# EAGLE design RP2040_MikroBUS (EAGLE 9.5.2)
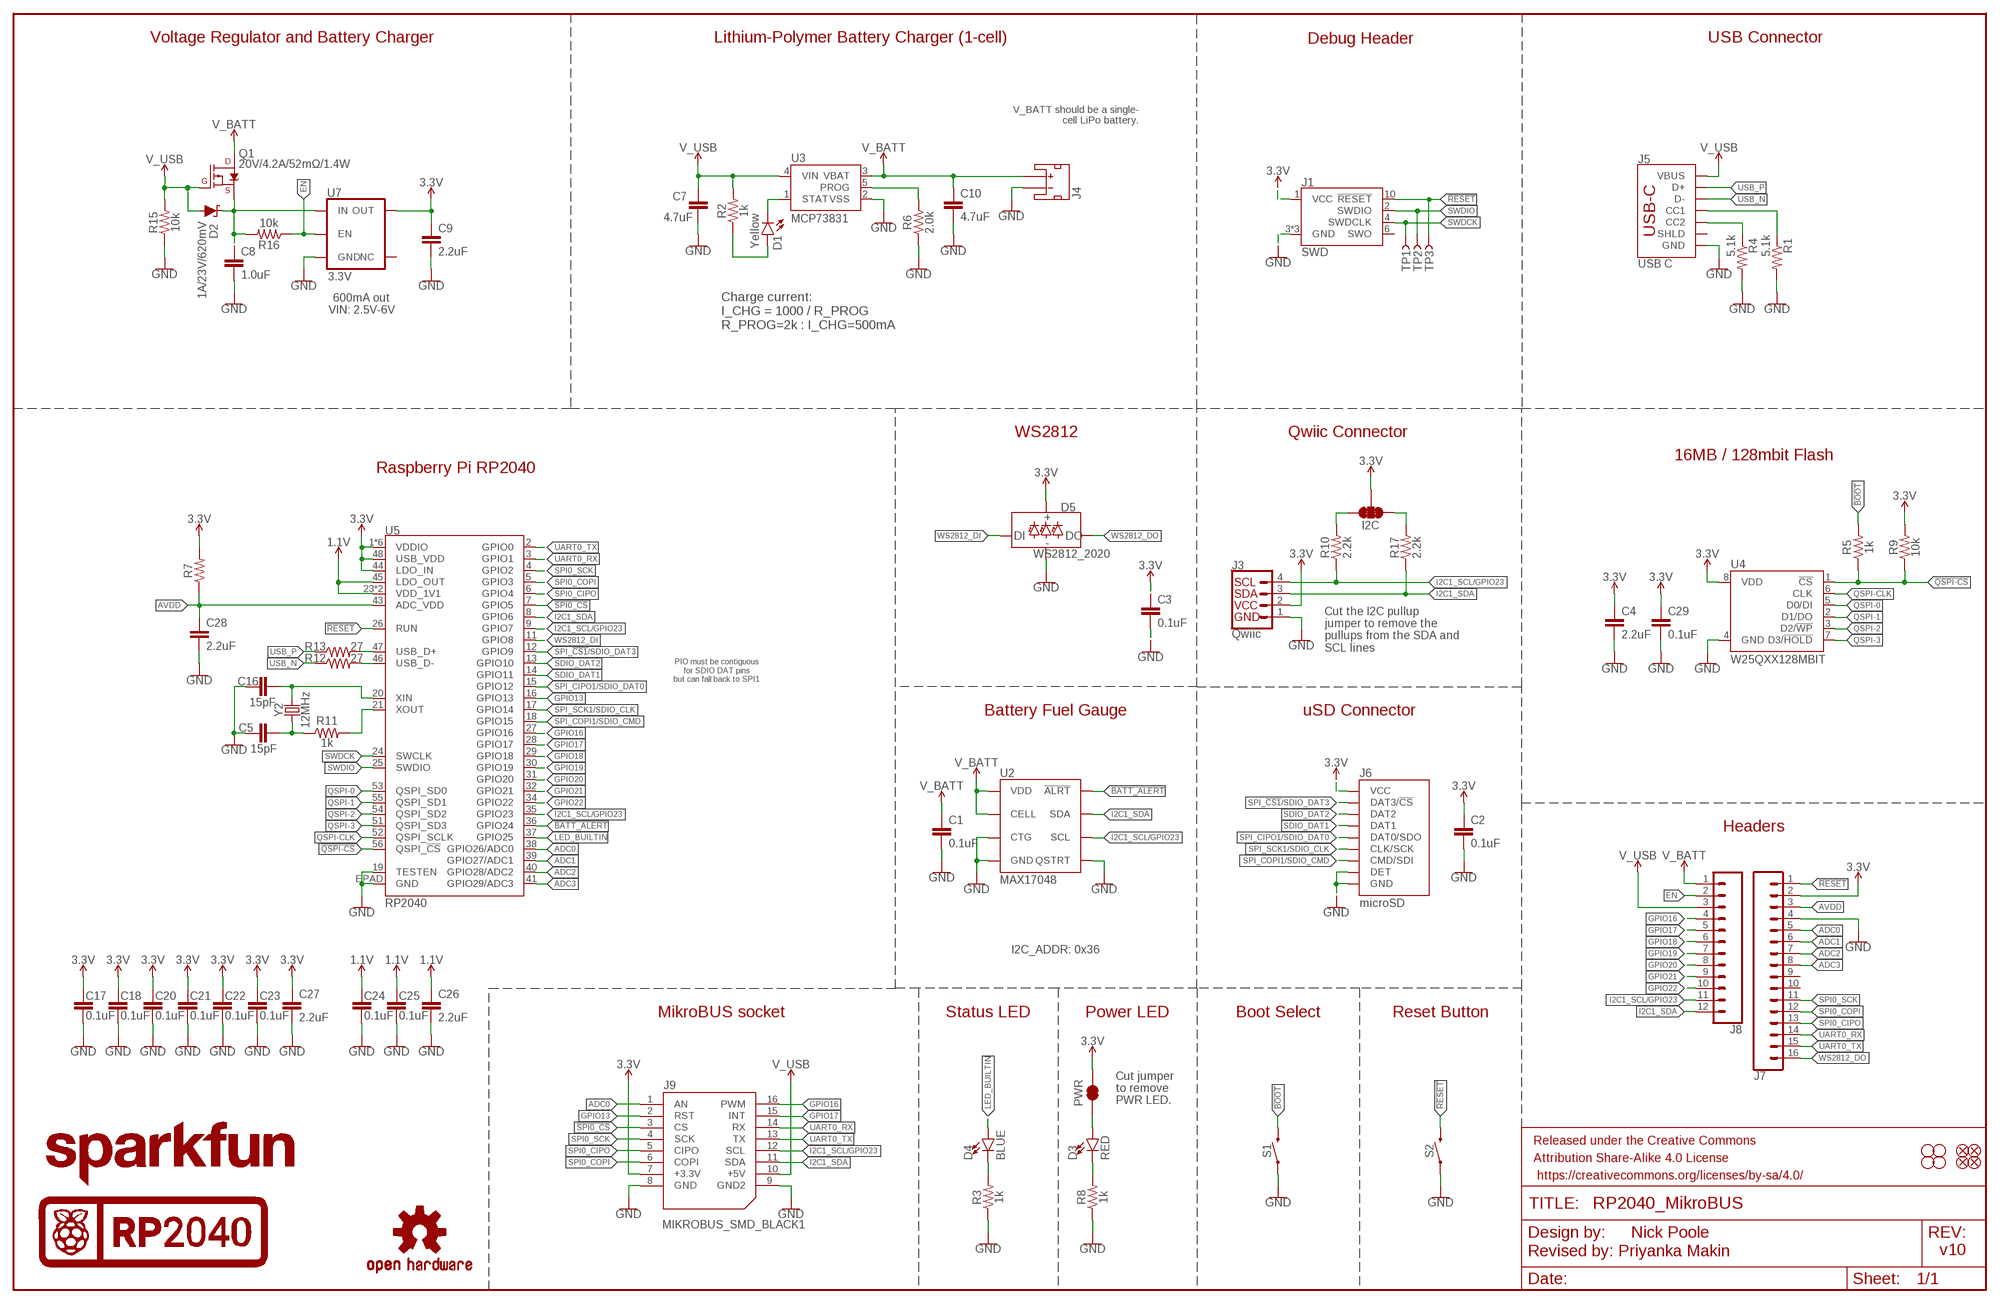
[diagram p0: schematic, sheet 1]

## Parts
C1  0.1uF  0.1UF-0402T-6.3V-10%-X7R  [0402-TIGHT]
C2  0.1uF  0.1UF-0402T-6.3V-10%-X7R  [0402-TIGHT]
C3  0.1uF  0.1UF-0402T-6.3V-10%-X7R  [0402-TIGHT]
C4  2.2uF  2.2UF-0402_TIGHT-10V-10%-X5R  [0402-TIGHT]
C5  15pF  15PF-0402T-50V-5%  [0402-TIGHT]
C7  4.7uF  4.7UF-0402_TIGHT-6.3V-20%-X5R  [0402-TIGHT]
C8  1.0uF  1.0UF-0402T-16V-10%  [0402-TIGHT]
C9  2.2uF  2.2UF-0402_TIGHT-10V-10%-X5R  [0402-TIGHT]
C10  4.7uF  4.7UF-0402_TIGHT-6.3V-20%-X5R  [0402-TIGHT]
C16  15pF  15PF-0402T-50V-5%  [0402-TIGHT]
C17  0.1uF  0.1UF-0402T-6.3V-10%-X7R  [0402-TIGHT]
C18  0.1uF  0.1UF-0402T-6.3V-10%-X7R  [0402-TIGHT]
C20  0.1uF  0.1UF-0402T-6.3V-10%-X7R  [0402-TIGHT]
C21  0.1uF  0.1UF-0402T-6.3V-10%-X7R  [0402-TIGHT]
C22  0.1uF  0.1UF-0402T-6.3V-10%-X7R  [0402-TIGHT]
C23  0.1uF  0.1UF-0402T-6.3V-10%-X7R  [0402-TIGHT]
C24  0.1uF  0.1UF-0402T-6.3V-10%-X7R  [0402-TIGHT]
C25  0.1uF  0.1UF-0402T-6.3V-10%-X7R  [0402-TIGHT]
C26  2.2uF  2.2UF-0402_TIGHT-10V-10%-X5R  [0402-TIGHT]
C27  2.2uF  2.2UF-0402_TIGHT-10V-10%-X5R  [0402-TIGHT]
C28  2.2uF  2.2UF-0402_TIGHT-10V-10%-X5R  [0402-TIGHT]
C29  0.1uF  0.1UF-0402T-6.3V-10%-X7R  [0402-TIGHT]
D1  Yellow  LED-YELLOW0603  [LED-0603]
D2  1A/23V/620mV  DIODE-SCHOTTKY-BAT20J  [SOD-323]
D3  RED  LED-RED0603  [LED-0603]
D4  BLUE  LED-BLUE0603  [LED-0603]
D5  WS2812_2020  [WS2812-2020]
FD1  FIDUCIALUFIDUCIAL  [FIDUCIAL-MICRO]
FD2  FIDUCIALUFIDUCIAL  [FIDUCIAL-MICRO]
FD3  FIDUCIALUFIDUCIAL  [FIDUCIAL-MICRO]
FD4  FIDUCIALUFIDUCIAL  [FIDUCIAL-MICRO]
FRAME1  FRAME-LEDGER  [CREATIVE_COMMONS]
H1  STAND-OFF  [STAND-OFF]
H2  STAND-OFF  [STAND-OFF]
H3  STAND-OFF  [STAND-OFF]
H4  STAND-OFF  [STAND-OFF]
I2C  JUMPER-SMT_3_2-NC_TRACE_SILK  [SMT-JUMPER_3_2-NC_TRACE_SILK]
J1  SWD  CORTEX_JTAG_DEBUG_MINIMUM_PTH  [2X5-PTH-1.27MM]
J3  Qwiic  QWIIC_CONNECTORJS-1MM  [JST04_1MM_RA]
J4  JST_2MM_MALE  [JST-2-SMD]
J5  USB C  USB_C_4-LAYER-ISOLATED  [USB-C-16P-4LAYER-ISOLATED]
J6  microSD  MICRO-SD-PUSH-PUSH-EXT-PIN  [MICROSD-EXTERNALPIN]
J7  CONN_161X16_NO_SILK  [1X16_NO_SILK]
J8  CONN_12NO_SILK  [1X12_NO_SILK]
J9  MIKROBUS_SMD_BLACK1  [MIKROBUS_SMD_BLACK]
LOGO1  OSHW-LOGOS  [OSHW-LOGO-S]
LOGO2  SFE_LOGO_NAME.1_INCH  [SFE_LOGO_NAME_.1]
PWR  JUMPER-SMT_2_NC_TRACE_SILK  [SMT-JUMPER_2_NC_TRACE_SILK]
Q1  20V/4.2A/52mΩ/1.4W  MOSFET_PCH-DMG2305UX-7  [SOT23-3]
R1  5.1k  5.1KOHM-0402T-1/16W-1%  [0402-TIGHT]
R2  1k  1KOHM-0402T-1/16W-1%  [0402-TIGHT]
R3  1k  1KOHM-0402T-1/16W-1%  [0402-TIGHT]
R4  5.1k  5.1KOHM-0402T-1/16W-1%  [0402-TIGHT]
R5  1k  1KOHM-0402T-1/16W-1%  [0402-TIGHT]
R6  2.0k  2.0KOHM-0603-1/10W-5%  [0603]
R7  200OHM-0402T-1/16W-1%  [0402-TIGHT]
R8  1k  1KOHM-0402T-1/16W-1%  [0402-TIGHT]
R9  10k  10KOHM-0402T-1/16W-1%  [0402-TIGHT]
R10  2.2k  2.2KOHM-0402T-1/16W-1%  [0402-TIGHT]
R11  1k  1KOHM-0402T-1/16W-1%  [0402-TIGHT]
R12  27  27OHM  [0402-TIGHT]
R13  27  27OHM  [0402-TIGHT]
R15  10k  10KOHM-0402T-1/16W-1%  [0402-TIGHT]
R16  10k  10KOHM-0402T-1/16W-1%  [0402-TIGHT]
R17  2.2k  2.2KOHM-0402T-1/16W-1%  [0402-TIGHT]
S1  MOMENTARY-SWITCH-SPST-SMD-5.2MM-TALL  [TACTILE_SWITCH_SMD_5.2MM]
S2  MOMENTARY-SWITCH-SPST-SMD-5.2MM-TALL  [TACTILE_SWITCH_SMD_5.2MM]
TP1  TEST-POINT3X4  [PAD.03X.04]
TP2  TEST-POINT3X4  [PAD.03X.04]
TP3  TEST-POINT3X4  [PAD.03X.04]
U2  MAX17048  MAX17048DFN8  [DFN-8]
U3  MCP73831  [SOT23-5]
U4  W25QXX128MBIT  W25QXX128MBIT-6X5-SKINNY_CENTER  [WSON-8-6X5-SKINNY_CENTERPAD]
U5  RP2040  [QFN-56]
U7  3.3V  V_REG_AP2112K-3.3V  [SOT23-5]
U$17  RASPI_RP2040_LOGO_10MM  [RASPI_RP2040_LOGO_10MM]
U$73  RASPI_RP2040_LOGO_10MM  [RASPI_RP2040_LOGO_10MM]
Y2  12MHz  CRYSTAL-12MHZ  [CRYSTAL-SMD-2X2.5MM]

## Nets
1.1V: C24.1 C25.1 C26.1 U5.23(VDD_1V1) U5.45(LDO_OUT) U5.50(VDD_1V1)
3.3V: C2.1 C3.1 C4.1 C9.1 C17.1 C18.1 C20.1 C21.1 C22.1 C23.1 C27.1 C29.1 D5.VCC I2C.2 J1.1(VCC) J3.2 J6.4(VCC) J7.2 J9.7(+3.3V) PWR.2 R7.2 R9.2 U4.8(VDD) U5.1(VDDIO) U5.10(VDDIO) U5.22(VDDIO) U5.33(VDDIO) U5.42(VDDIO) U5.44(LDO_IN) U5.48(USB_VDD) U5.49(VDDIO) U7.5(OUT)
!BATT_ALERT!: U2.5(!ALRT) U5.36(GPIO24)
!BOOT!: R5.2 S1.3
!QSPI-CS!: R5.1 R9.1 U4.1(!CS!) U5.56(QSPI_!CS!)
!RESET!: J1.10(!RESET) J7.1 S2.3 TP3.1 U5.26(RUN)
!SPI0_CS!: J9.3(CS) U5.7(GPIO5)
ADC0: J7.5 J9.1(AN) U5.38(GPIO26/ADC0)
ADC1: J7.6 U5.39(GPIO27/ADC1)
ADC2: J7.7 U5.40(GPIO28/ADC2)
ADC3: J7.8 U5.41(GPIO29/ADC3)
AVDD: C28.1 J7.3 R7.1 U5.43(ADC_VDD)
EN: J8.2 R16.1 U7.3(EN)
GND: C1.2 C2.2 C3.2 C4.2 C5.1 C7.2 C8.2 C9.2 C10.2 C16.1 C17.2 C18.2 C20.2 C21.2 C22.2 C23.2 C24.2 C25.2 C26.2 C27.2 C28.2 C29.2 D5.GND J1.3(GND) J1.5(GND) J1.9(GND) J3.1 J4.1(-) J5.GND J5.GND2(GND) J6.6(GND) J6.9(DET) J6.10(GND) J6.11(GND) J6.12(GND) J6.13(GND) J7.4 J9.8(GND) J9.9(GND2) R1.2 R3.1 R4.2 R6.1 R8.1 R15.1 S1.1 S2.1 U2.1(CTG) U2.4(GND) U2.6(QSTRT) U2.9(GND) U3.2(VSS) U4.4(GND) U5.19(TESTEN) U5.EPAD(GND) U7.2(GND)
GPIO13: J9.2(RST) U5.16(GPIO13)
GPIO16: J8.4 J9.16(PWM) U5.27(GPIO16)
GPIO17: J8.5 J9.15(INT) U5.28(GPIO17)
GPIO18: J8.6 U5.29(GPIO18)
GPIO19: J8.7 U5.30(GPIO19)
GPIO20: J8.8 U5.31(GPIO20)
GPIO21: J8.9 U5.32(GPIO21)
GPIO22: J8.10 U5.34(GPIO22)
I2C1_SCL/GPIO23: J3.4 J8.11 J9.12(SCL) R10.1 U2.7(SCL) U5.9(GPIO7) U5.35(GPIO23)
I2C1_SDA: J3.3 J8.12 J9.11(SDA) R17.1 U2.8(SDA) U5.8(GPIO6)
LED_BUILTIN: D4.A U5.37(GPIO25)
N$1: D4.C R3.2
N$2: I2C.3 R10.2
N$3: I2C.1 R17.2
N$4: R11.2 U5.21(XOUT)
N$5: C16.2 U5.20(XIN) Y2.P3
N$6: C5.2 R11.1 Y2.P1
N$7: D3.C R8.2
N$9: D1.C U3.1(STAT)
N$10: D3.A PWR.1
N$11: J5.A5(CC1) R1.1
N$12: J5.B5(CC2) R4.1
N$14: R6.2 U3.5(PROG)
N$15: C8.1 D2.C Q1.2(S) R16.2 U7.1(IN)
N$17: D1.A R2.1
QSPI-0: U4.5(D0/DI) U5.53(QSPI_SD0)
QSPI-1: U4.2(D1/DO) U5.55(QSPI_SD1)
QSPI-2: U4.3(D2/!WP!) U5.54(QSPI_SD2)
QSPI-3: U4.7(D3/!HOLD!) U5.51(QSPI_SD3)
QSPI-CLK [Clock]: U4.6(CLK) U5.52(QSPI_SCLK)
SDIO_DAT1: J6.8(DAT1) U5.14(GPIO11)
SDIO_DAT2: J6.1(DAT2) U5.13(GPIO10)
SPI0_CIPO: J7.13 J9.5(CIPO) U5.6(GPIO4)
SPI0_COPI: J7.12 J9.6(COPI) U5.5(GPIO3)
SPI0_SCK: J7.11 J9.4(SCK) U5.4(GPIO2)
SPI_!CS1!/SDIO_DAT3: J6.2(DAT3/!CS!) U5.12(GPIO9)
SPI_CIPO1/SDIO_DAT0: J6.7(DAT0/SDO) U5.15(GPIO12)
SPI_COPI1/SDIO_CMD: J6.3(CMD/SDI) U5.18(GPIO15)
SPI_SCK1/SDIO_CLK: J6.5(CLK/SCK) U5.17(GPIO14)
SWDCK: J1.4(SWDCLK) TP1.1 U5.24(SWCLK)
SWDIO: J1.2(SWDIO) TP2.1 U5.25(SWDIO)
UART0_RX: J7.14 J9.14(RX) U5.3(GPIO1)
UART0_TX: J7.15 J9.13(TX) U5.2(GPIO0)
USB_F_N: R12.2 U5.46(USB_D-)
USB_F_P: R13.2 U5.47(USB_D+)
USB_N: J5.A7(D-) J5.B7(D-) R12.1
USB_P: J5.A6(D+) J5.B6(D+) R13.1
V_BATT: C1.1 C10.1 J4.2(+) J8.1 Q1.3(D) U2.2(CELL) U2.3(VDD) U3.3(VBAT)
V_USB: C7.1 D2.A J5.VBUS1(VBUS) J5.VBUS2(VBUS) J8.3 J9.10(+5V) Q1.1(G) R2.2 R15.2 U3.4(VIN)
WS2812_DI: D5.DI U5.11(GPIO8)
WS2812_DO: D5.DO J7.16
Unconnected: J1.6(SWO) J4.NC1(PAD1) J4.NC2(PAD2) J5.SHLD1(SHLD) J5.SHLD2(SHLD) J5.SHLD3(SHLD) J5.SHLD4(SHLD) J5.SHLD5(SHLD) J5.SHLD6(SHLD) J5.SHLD7(SHLD) J5.SHLD8(SHLD) J7.9 J7.10 U7.4(NC)

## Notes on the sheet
- Voltage Regulator and Battery Charger | Lithium-Polymer Battery Charger (1-cell) | Debug Header | USB Connector
- V_BATT should be a single-
  cell LiPo battery.
- Charge current:
  I_CHG = 1000 / R_PROG
  R_PROG=2k : I_CHG=500mA
- 600mA out
  VIN: 2.5V-6V
- WS2812 | Qwiic Connector
- 16MB / 128mbit Flash
- Raspberry Pi RP2040
- Cut the I2C pullup 
  jumper to remove the 
  pullups from the SDA and 
  SCL lines
- PIO must be contiguous
  for SDIO DAT pins
  but can fall back to SPI1
- Battery Fuel Gauge | uSD Connector
- Headers
- I2C_ADDR: 0x36
- MikroBUS socket | Status LED | Power LED | Boot Select | Reset Button
- Cut jumper
  to remove
  PWR LED.
- Nick Poole
- v10
- Revised by: Priyanka Makin

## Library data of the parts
C1-C3 C17 C18 C20-C25 C29 = SparkFun-Capacitors:0.1UF: 0.1µF ceramic capacitors; PROD_ID: CAP-14993
C4 C9 C26-C28 = SparkFun-Capacitors:2.2UF: 2.2µF ceramic capacitors; PROD_ID: CAP-14232
C5 C16 = SparkFun-Capacitors:15PF: 15pF ceramic capacitors; PROD_ID: CAP-13063
C7 C10 = SparkFun-Capacitors:4.7UF: 4.7µF ceramic capacitors; PROD_ID: CAP-14240
C8 = SparkFun-Capacitors:1.0UF: 1µF ceramic capacitors; PROD_ID: CAP-12417
D1 = SparkFun-LED:LED-YELLOW: Yellow SMD LED; PROD_ID: DIO-09003
D2 = SparkFun-DiscreteSemi:DIODE-SCHOTTKY: Schottky diode; PROD_ID: DIO-11623
D3 = SparkFun-LED:LED-RED: Red SMD LED; PROD_ID: DIO-00819
D4 = SparkFun-LED:LED-BLUE: Blue SMD LED; PROD_ID: DIO-08575
D5 = SparkFun-LED:WS2812: Addressable RGB LED - 1 Wire Common names: WS2812, SK6812, Neopixel, APA-106, etc. SMD LED with built-in controller IC. Color: Red/Green/Blue SparkFun Products: LED-SMD RGB (WS2812) LED - RGB Addressable, PTH, 5mm Diffused (5 Pack) LED - RGB Addressable, PTH, 5mm Clear (5 Pack) Blynk Board -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; PROD_ID: DIO-15591
FD1-FD4 = SparkFun-Aesthetics:FIDUCIAL: Fiducial Alignment Points
FRAME1 = SparkFun-Aesthetics:FRAME-LEDGER: Schematic Frame - Ledger
H1-H4 = SparkFun-Hardware:STAND-OFF: Stand Off
I2C = SparkFun-Jumpers:JUMPER-SMT_3_2-NC_TRACE: Normally closed trace jumper (2 of 2 connections) This jumper has a trace between all three pads so they are normally closed (NC). Use a razor knife to open the connection(s). For best results follow the IPC guidelines for cutting traces: Cutout at least 0.063 mm (0.005 in). Remove all loose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
J1 = SparkFun-Connectors:CORTEX_JTAG_DEBUG_MINIMUM: Cortex Debug Connector - 10 pin Supports JTAG debug, Serial Wire debug, and Serial Wire Viewer. PTH and SMD connector options available. General Connector Information Products: PTH Connector -via Digi-Key SparkFun PSoc SparkFun T
J3 = SparkFun-Connectors:QWIIC_CONNECTOR: SparkFun I2C Standard Qwiic Connector An SMD 1mm pitch JST connector makes it easy and quick (get it? Qwiic?) to connect I2C devices to each other. The Qwiic system enables fast and solderless connection between popular platforms and various sensors and actuators. We carry 200mm, 100mm, 50mm, and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; PROD_ID: CONN-13694; VALUE: QWIIC_RIGHT_ANGLE
J4 = SparkFun-Connectors:JST_2MM_MALE: JST 2MM MALE RA CONNECTOR Two pin, compact surface mount connector. Commonly used as a battery input connection point. We really like the solid locking feeling and high current rating on these small connectors. We use these all the time as battery connectors. Mates to single-cell LiPo batteries.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; PROD_ID: CONN-11443; SF_ID: PRT-08612
J5 = SparkFun-Connectors:USB_C: USB Type C 16Pin Connector Super Speed pins not available on the 16-pin purely SMD connector so this part is best for USB 2.0 implementations. D1 and D2 are tied together enabling D+/- no matter which way the cable is plugged into the connector. The two channel configuration pins (CC1/2) are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; PROD_ID: CONN-14122; VALUE: USB Female Type C Connector
J6 = SparkFun-Connectors:MICRO-SD: microSD Socket for Transflash Various sockets for µSD. tDoc lines correctly indicate media card edge positions when inserting (unlocked, locked, depressed). NOTE: CD1 and CD2 are connected internally, and the default detect state of the socket is detect pin to ground. SparkFun Products: WAV Trigger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; PROD_ID: CONN-16110
J7 = SparkFun-Connectors:CONN_16: Multi connection point. Often used as Generic Header-pin footprint for 0.1 inch spaced/style header connections On any of the 0.1 inch spaced packages, you can populate with these: Break Away Headers - Straight (PRT-00116) Break Away Male Headers - Right Angle (PRT-00553) Female Headers (PRT-00115)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
J8 = SparkFun-Connectors:CONN_12: Multi connection point. Often used as Generic Header-pin footprint for 0.1 inch spaced/style header connections On any of the 0.1 inch spaced packages, you can populate with these: Break Away Headers - Straight (PRT-00116) Break Away Male Headers - Right Angle (PRT-00553) Female Headers (PRT-00115)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
J9 = mikroBUS_SMD_BLACK:MIKROBUS_SMD_BLACK; PROD_ID: CONN-16267
LOGO1 = SparkFun-Aesthetics:OSHW-LOGO: Open-Source Hardware (OSHW) Logo
LOGO2 = SparkFun-Aesthetics:SFE_LOGO_NAME: SparkFun Font Logo
PWR = SparkFun-Jumpers:JUMPER-SMT_2_NC_TRACE: Normally closed trace jumper
Q1 = SparkFun-DiscreteSemi:MOSFET_PCH: P-channel MOSFETs Voltage controlled devices that allow control of high current outputs. SparkFun Products: SparkFun ESP32 Thing SparkFun ESP8266 Thing SparkFun Pi Servo HAT V2 DMG2305UX-7 (20V/4.2A/SOT23-3); PROD_ID: TRANS-14388
R1 R4 = SparkFun-Resistors:5.1KOHM; PROD_ID: RES-14340
R2 R3 R5 R8 R11 = SparkFun-Resistors:1KOHM: 1kΩ resistor; PROD_ID: RES-14342
R6 = SparkFun-Resistors:2.0KOHM: 2kΩ resistor; PROD_ID: RES-08296
R7 = SparkFun-Resistors:200OHM: 200Ω resistor; PROD_ID: RES-15550
R9 R15 R16 = SparkFun-Resistors:10KOHM: 10kΩ resistor; PROD_ID: RES-14241
R10 R17 = SparkFun-Resistors:2.2KOHM: 2.2kΩ resistor; PROD_ID: RES-14341
R12 R13 = SparkFun-Resistors:27OHM: 27Ω resistor; PROD_ID: RES-15238
S1 S2 = SparkFun-Switches:MOMENTARY-SWITCH-SPST: Momentary Switch (Pushbutton) - SPST; PROD_ID: SWCH-14139
TP1-TP3 = SparkFun-Connectors:TEST-POINT: SparkFun Test Points
U2 = SparkFun-IC-Power:MAX17048: Micropower 1-Cell Li+ ModelGauge SparkFun Products Qduino Mini (DEV-13614); PROD_ID: IC-12551
U3 = SparkFun-IC-Power:MCP73831: MCP73831T Li-Ion, Li-Pol Controller Miniature single cell, fully integrated Li-Ion, Li-polymer charge management controller Datasheet SparkFun Products: SparkFun ESP32 Thing SparkFun 9DoF Razor IMU M0; PROD_ID: IC-09995
U4 = SparkFun-IC-Memory:W25QXX; PROD_ID: IC-15107
U5 = SparkFun-IC-Microcontroller:RP2040: Raspberry Pi RP2040 MCU 56-pin 32-bit Microcontroller with 264kB of SRAM and external flash support up to 16MB Getting Started with the RP2040 Dual-core ARM Cortex M0+ processor, flexible clock running up to 133 MHz 264kB of SRAM, and QSPI control of common flash memory USB 1.1 Host and Device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; PROD_ID: IC-15502
U7 = SparkFun-IC-Power:V_REG_AP2112: AP2112 - 600mA CMOS LDO Regulator w/ Enable The AP2112 is CMOS process low dropout linear regulator with enable function, the regulator delivers a guaranteed 600mA (min.) continuous load current. Features Output Voltage Accuracy: ±1.5% Output Current: 600mA (Min.) Foldback Short Current Protection: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; PROD_ID: VREG-12457
U$17 U$73 = SparkFun-Aesthetics:RASPI_RP2040_LOGO
Y2 = SparkFun-Clocks:CRYSTAL-12MHZ: 12.0MHz Crystal; PROD_ID: XTAL-15540

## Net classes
0 default: width 0 mm, drill 0 mm
2 Clock: width 0.089 mm, clearance 0.178 mm

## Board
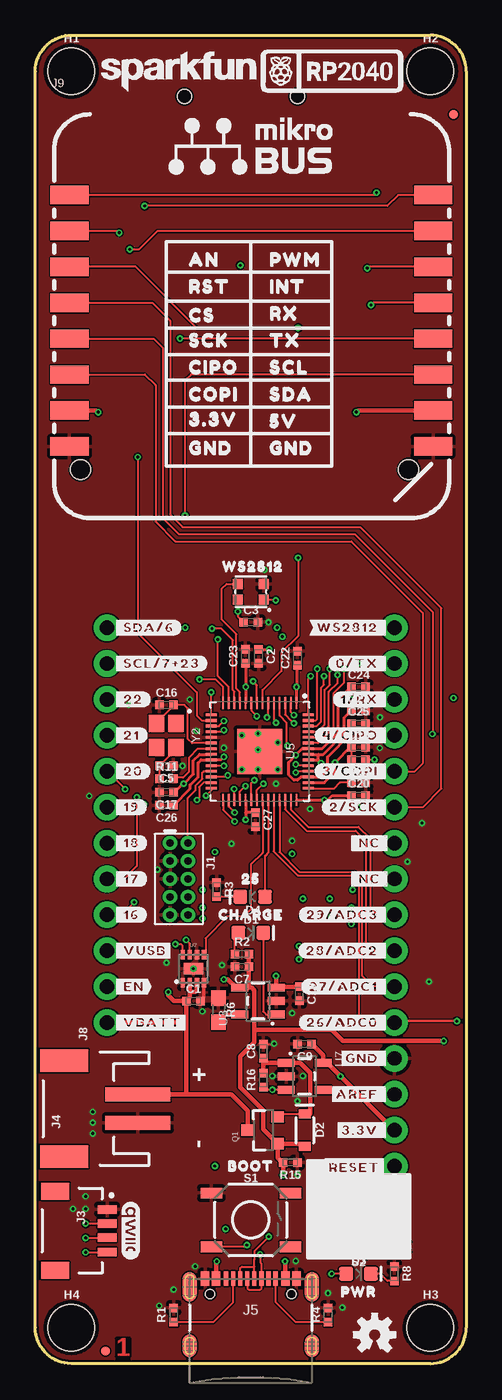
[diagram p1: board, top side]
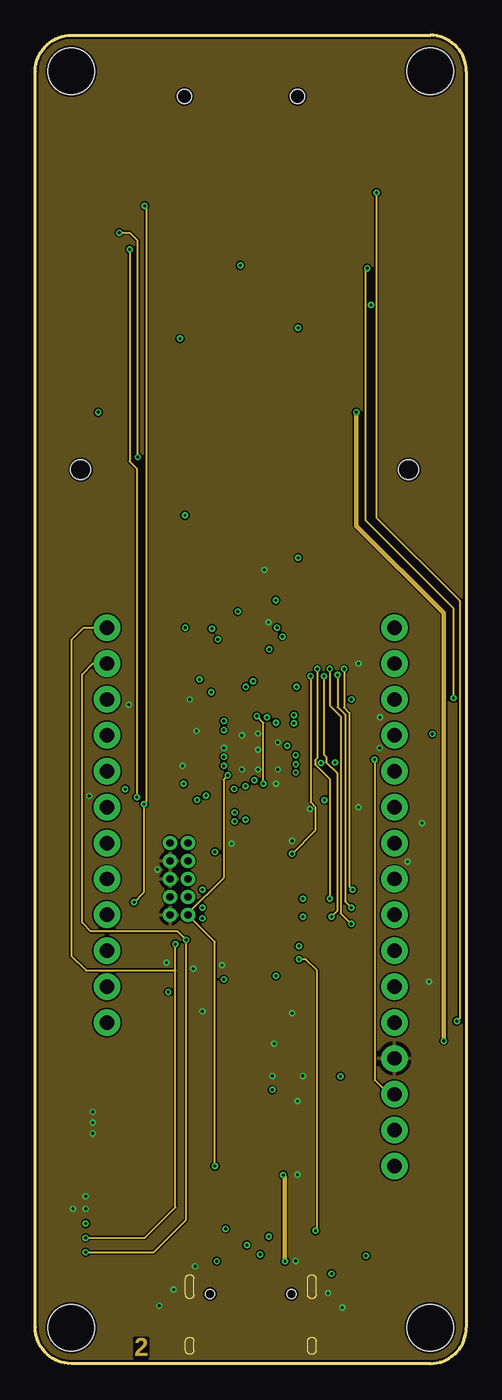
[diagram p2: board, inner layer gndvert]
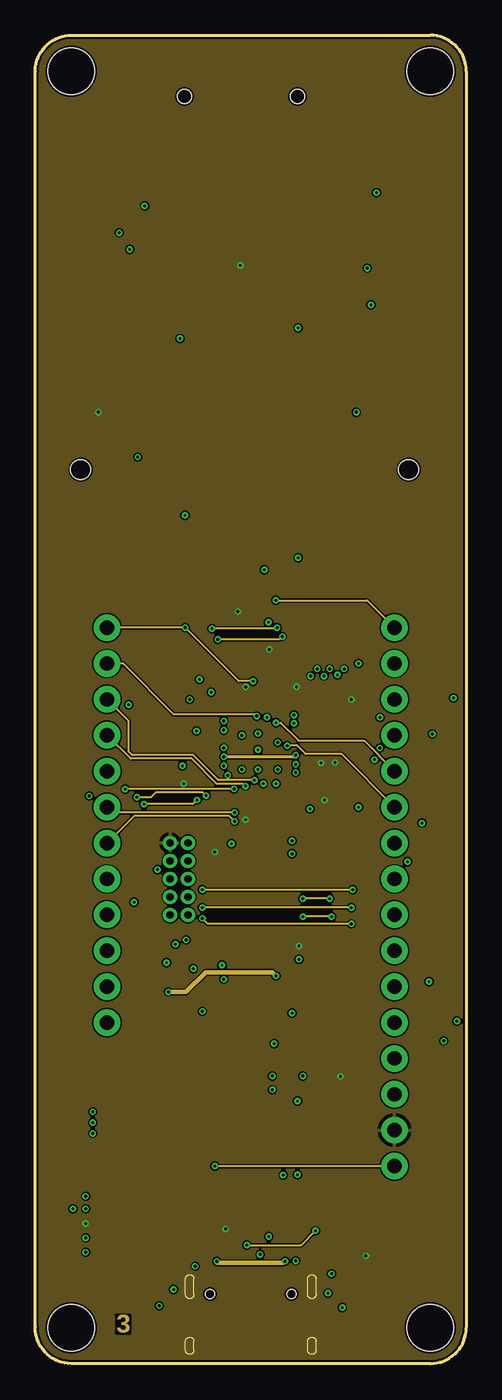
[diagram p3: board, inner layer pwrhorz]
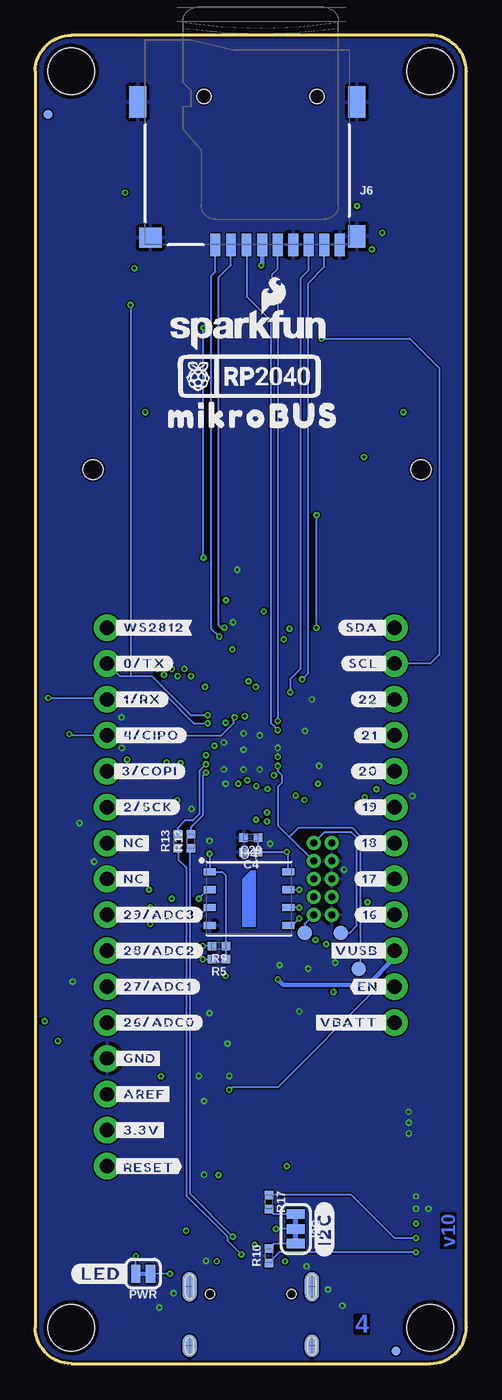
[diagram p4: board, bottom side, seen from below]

Size 30.48 x 93.98 mm. Coordinates in mm from the lower left corner, seen from the top.
Outline: 2.54,93.98 27.94,93.98 arc-90 30.48,91.44 30.48,2.54 arc-90 27.94,0 2.54,0 arc-90 0,2.54 0,91.44 arc-90 2.54,93.98
Copper layers (1+2*15+16): Top 0.035mm / dielectric 1.5mm / gndvert 0.035mm / dielectric 0.15mm / pwrhorz 0.035mm / dielectric 0.2mm / Bottom 0.035mm
Design rules "SparkFun-4-Layer-MicroMod-JLCPCB": minimum track width 4mil, minimum drill 0.2mm, track to track 4mil, track to pad 4mil, pad to pad 4mil, via to via 4mil, smd to smd 4mil, copper to edge 6mil, drill to drill 6mil, minimum pad ring 3mil, minimum via ring 3mil, stop-mask expansion 2.5mil, vias tented up to drill 25mil, thermal gap 10mil

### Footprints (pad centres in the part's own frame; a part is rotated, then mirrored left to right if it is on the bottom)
0402-TIGHT = smd 0.6 x 0.6: 1 -0.5,0; 2 0.5,0
LED-0603 = smd 1 x 1: A -0.877,0; C 0.877,0
SOD-323 = smd 0.63 x 0.83: A 1.15,0; C -1.15,0
WS2812-2020 = smd 0.7 x 0.7: DI -0.915,0.55; DO 0.915,-0.55; GND 0.915,0.55; VCC -0.915,-0.55
FIDUCIAL-MICRO = smd 0.635 x 0.635: 1 0,0
STAND-OFF = hole 3.302: 0,0
SMT-JUMPER_3_2-NC_TRACE_SILK = smd 0.66 x 1.27: 1 -1.041,0; 2 0,0; 3 1.041,0
2X5-PTH-1.27MM = drill 0.508 pad 1: 1 -2.54,-0.635; 2 -2.54,0.635; 3 -1.27,-0.635; 4 -1.27,0.635; 5 0,-0.635; 6 0,0.635; 7 1.27,-0.635; 8 1.27,0.635; 9 2.54,-0.635; 10 2.54,0.635
JST04_1MM_RA = smd 0.6 x 1.35: 1 -1.5,0; 2 -0.5,0; 3 0.5,0; 4 1.5,0 | smd 1.2 x 2: NC1 2.8,-3.675; NC2 -2.8,-3.675
JST-2-SMD = smd 1 x 4.6: 1 -1,-3.7; 2 1,-3.7 | smd 1.6 x 3.4: NC1 -3.4,1.5; NC2 3.4,1.5
USB-C-16P-4LAYER-ISOLATED = smd 0.3 x 1: A5 -1.25,-0.34; A6 -0.25,-0.34; A7 0.25,-0.34; A8 1.25,-0.34; B5 1.75,-0.34; B6 0.75,-0.34; B7 -0.75,-0.34; B8 -1.75,-0.34 | smd 0.6 x 1: GND -3.225,-0.34; GND2 3.225,-0.34; VBUS1 -2.45,-0.34; VBUS2 2.45,-0.34 | smd 1 x 2.1: SHLD1 -4.32,-0.915; SHLD2 4.32,-0.915 | smd 1 x 2.1 bottom: SHLD3 -4.32,-0.915; SHLD4 4.32,-0.915 | smd 1 x 1.6: SHLD5 -4.32,-5.095; SHLD8 4.32,-5.095 | smd 1 x 1.6 bottom: SHLD6 -4.32,-5.095; SHLD7 4.32,-5.095 | hole 0.65: -2.89,-1.445; 2.89,-1.445
MICROSD-EXTERNALPIN = smd 0.7 x 1.6: 1 2.25,10.5; 2 1.15,10.5; 3 0.05,10.5; 4 -1.05,10.5; 5 -2.15,10.5; 6 -3.25,10.5; 7 -4.35,10.5; 8 -5.45,10.5; 9 -6.55,10.5 | smd 1.2 x 1.6: 10 -7.75,9.9 | smd 1.2 x 2.2: 11 -7.75,0.4; 12 7.75,0.4 | smd 1.6 x 1.4: 13 6.85,10 | hole 1: 3.05,0; -4.95,0
1X16_NO_SILK = drill 1.016 pad 1.88: 1 0,0; 2 2.54,0; 3 5.08,0; 4 7.62,0; 5 10.16,0; 6 12.7,0; 7 15.24,0; 8 17.78,0; 9 20.32,0; 10 22.86,0; 11 25.4,0; 12 27.94,0; 13 30.48,0; 14 33.02,0; 15 35.56,0; 16 38.1,0
1X12_NO_SILK = drill 1.016 pad 1.88: 1 0,0; 2 2.54,0; 3 5.08,0; 4 7.62,0; 5 10.16,0; 6 12.7,0; 7 15.24,0; 8 17.78,0; 9 20.32,0; 10 22.86,0; 11 25.4,0; 12 27.94,0
MIKROBUS_SMD_BLACK = smd 2.7 x 1.3: 1 -12.7,8.89; 2 -12.7,6.35; 3 -12.7,3.81; 4 -12.7,1.27; 5 -12.7,-1.27; 6 -12.7,-3.81; 7 -12.7,-6.35; 8 -12.7,-8.89; 9 13.02,-8.89; 10 13.02,-6.35; 11 13.02,-3.81; 12 13.02,-1.27; 13 13.02,1.27; 14 13.02,3.81; 15 13.02,6.35; 16 13.02,8.89 | hole 1.4: -11.914,-10.541; 11.286,-10.541
SMT-JUMPER_2_NC_TRACE_SILK = smd 0.66 x 1.27: 1 -0.521,0; 2 0.521,0
SOT23-3 = smd 0.8 x 0.9: 1 -0.95,-1; 2 0.95,-1; 3 0,1.1
0603 = smd 1.1 x 1: 1 -0.85,0; 2 0.85,0
TACTILE_SWITCH_SMD_5.2MM = smd 1.524 x 0.762: 1 -2.794,1.905; 2 2.794,1.905; 3 -2.794,-1.905; 4 2.794,-1.905
PAD.03X.04 = smd 1.016 x 1.016: 1 0,0
DFN-8 = smd 0.3 x 0.7: 1 -0.75,-0.99; 2 -0.25,-0.99; 3 0.25,-0.99; 4 0.75,-0.99; 5 0.75,0.99; 6 0.25,0.99; 7 -0.25,0.99; 8 -0.75,0.99 | smd 1.38 x 0.8: 9 0,0
SOT23-5 = smd 0.55 x 1.2: 1 -0.95,-1.3; 2 0,-1.3; 3 0.95,-1.3; 4 0.95,1.3; 5 -0.95,1.3
WSON-8-6X5-SKINNY_CENTERPAD = smd 0.85 x 0.5: 1 -2.775,1.905; 2 -2.775,0.635; 3 -2.775,-0.635; 4 -2.775,-1.905; 5 2.775,-1.905; 6 2.775,-0.635; 7 2.775,0.635; 8 2.775,1.905
QFN-56 = smd 0.875 x 0.2: 1 -3.437,2.6; 2 -3.437,2.2; 3 -3.437,1.8; 4 -3.437,1.4; 5 -3.437,1; 6 -3.437,0.6; 7 -3.437,0.2; 8 -3.437,-0.2; 9 -3.437,-0.6; 10 -3.437,-1; 11 -3.437,-1.4; 12 -3.437,-1.8; 13 -3.437,-2.2; 14 -3.437,-2.6; 29 3.437,-2.6; 30 3.437,-2.2; 31 3.437,-1.8; 32 3.437,-1.4; 33 3.437,-1; 34 3.437,-0.6; 35 3.437,-0.2; 36 3.437,0.2; 37 3.437,0.6; 38 3.437,1; 39 3.437,1.4; 40 3.437,1.8; 41 3.437,2.2; 42 3.437,2.6 | smd 0.2 x 0.875: 15 -2.6,-3.437; 16 -2.2,-3.437; 17 -1.8,-3.437; 18 -1.4,-3.437; 19 -1,-3.437; 20 -0.6,-3.437; 21 -0.2,-3.437; 22 0.2,-3.437; 23 0.6,-3.437; 24 1,-3.437; 25 1.4,-3.437; 26 1.8,-3.437; 27 2.2,-3.437; 28 2.6,-3.437; 43 2.6,3.437; 44 2.2,3.437; 45 1.8,3.437; 46 1.4,3.437; 47 1,3.437; 48 0.6,3.437; 49 0.2,3.437; 50 -0.2,3.437; 51 -0.6,3.437; 52 -1,3.437; 53 -1.4,3.437; 54 -1.8,3.437; 55 -2.2,3.437; 56 -2.6,3.437 | smd 3.2 x 3.2: EPAD 0,0
CRYSTAL-SMD-2X2.5MM = smd 1.2 x 1.1: P1 0.846,0.69; P2 -0.854,0.69; P3 -0.854,-0.71; P4 0.846,-0.71

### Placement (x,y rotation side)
C1  11.18,25.65 0 top
C2  15.79,50.04 270 top
C3  15.24,52.45 0 top
C4  15.24,36.2 180 bottom
C5  9.27,42.29 180 top
C7  14.61,28.07 180 top
C8  16.13,22.1 90 top
C9  19.05,22.61 180 top
C10  18.67,26.16 270 top
C16  9.27,46.61 0 top
C17  9.27,40.42 180 top
C18  22.86,43.62 0 top
C20  22.86,40.18 0 top
C21  22.86,46.19 0 top
C22  18.54,49.91 90 top
C23  14.86,50.04 90 top
C24  22.86,47.88 0 top
C25  22.86,45.28 0 top
C26  9.27,39.5 180 top
C27  15.57,38.48 270 top
C28  22.86,41.1 0 top
C29  15.24,37.21 180 bottom
D1  15.24,30.48 0 top
D2  19.05,16.51 270 top
D3  22.86,6.35 0 top
D4  15.37,33.02 180 top
D5  15.24,54.61 0 top
FD1  4.95,0.89 0 top
FD2  29.59,88.39 0 top
FD3  4.95,0.89 0 bottom
FD4  29.59,88.39 0 bottom
FRAME1  not placed on the board
H1  2.54,91.44 0 top
H2  27.94,91.44 0 top
H3  27.94,2.54 0 top
H4  2.54,2.54 0 top
I2C  12.06,9.53 270 bottom
J1  10.16,34.29 270 top
J3  5.08,9.4 270 top
J4  3.56,18.03 90 top
J5  15.24,6.35 0 top
J6  15.49,89.66 180 bottom
J7  25.4,13.97 90 top
J8  5.08,24.13 90 top
J9  15.11,73.79 0 top
LOGO1  24,2.03 0 top
LOGO2  10.16,91.44 0 top
PWR  22.86,6.35 180 bottom
Q1  16.13,16.51 90 top
R1  9.78,3.43 90 top
R2  14.61,28.98 0 top
R3  12.83,33.53 270 top
R4  20.7,3.43 90 top
R5  17.5,28.61 180 bottom
R6  12.95,25.02 270 top
R7  22.86,42.71 180 top
R8  25.4,6.35 270 top
R9  17.5,29.54 180 bottom
R10  13.97,7.62 90 bottom
R11  9.27,41.36 0 top
R12  19.48,36.96 90 bottom
R13  20.42,36.96 90 bottom
R15  18.03,14.22 180 top
R16  16.13,20.07 90 top
R17  13.97,11.43 270 bottom
S1  15.24,10.16 0 top
S2  22.86,10.16 180 top
TP1  7.62,27.94 0 bottom
TP2  8.89,30.48 0 bottom
TP3  11.43,30.48 0 bottom
U2  11.18,27.94 0 top
U3  15.75,25.65 90 top
U4  15.37,32.89 0 bottom
U5  15.88,43.31 270 top
U7  19.05,20.32 270 top
U$1  [#_16#0]  5.46,31.75 0 top
U$2  [#_17#0]  5.46,34.29 0 top
U$3  [#_18#0]  5.46,36.83 0 top
U$4  [#_19#0]  5.46,39.37 0 top
U$5  [#_20#0]  5.46,41.91 0 top
U$6  [#_21#0]  5.46,44.45 0 top
U$7  [#_22#0]  5.46,46.99 0 top
U$8  [#_SCL#7#23#0]  5.46,49.53 0 top
U$9  [#_SDA#6#0]  5.46,52.07 0 top
U$10  [#WS2812_#0]  25.02,52.07 0 top
U$11  [#0#TX_#0]  25.02,49.53 0 top
U$12  [#1#RX_#0]  25.02,46.99 0 top
U$13  [#4#CIPO_#0]  25.02,44.45 0 top
U$14  [#3#COPI_#0]  25.02,41.91 0 top
U$15  [#2#SCK_#0]  25.02,39.37 0 top
U$16  [PWR0]  22.86,5.08 0 top
U$17  15.37,69.85 0 bottom
U$18  [#29#ADC3_#0]  25.02,31.75 0 top
U$19  [#28#ADC2_#0]  25.02,29.21 0 top
U$20  [#27#ADC1_#0]  25.02,26.67 0 top
U$21  [#26#ADC0_#0]  25.02,24.13 0 top
U$22  [#_VUSB#0]  5.46,29.21 0 top
U$23  [#_EN#0]  5.46,26.67 0 top
U$24  [#_VBATT#0]  5.46,24.13 0 top
U$25  [#GND_#0]  25.02,21.59 0 top
U$26  [#AREF_#0]  25.02,19.05 0 top
U$27  [#3#3V_#0]  25.02,16.51 0 top
U$28  [##RESET##0]  24.89,13.97 0 top
U$29  [AN0]  10.16,78.11 0 top
U$30  [WS28120]  12.7,56.39 0 top
U$31  [ORDERING_INSTRUCTIONS]  not placed on the board
U$32  [SFE_LOGO_NAME_FLAME_.1]  15.37,73.15 0 bottom
U$33  [#SCL_#0]  5.46,49.53 0 bottom
U$34  [#SDA_#0]  5.46,52.07 0 bottom
U$35  [#_#RESET##0]  25.02,13.97 0 bottom
U$36  [#_3#3V#0]  25.02,16.51 0 bottom
U$37  [#_AREF#0]  25.02,19.05 0 bottom
U$38  [#_GND#0]  25.02,21.59 0 bottom
U$39  [#_26#ADC0#0]  25.02,24.13 0 bottom
U$40  [#_27#ADC1#0]  25.02,26.67 0 bottom
U$41  [#_28#ADC2#0]  25.02,29.21 0 bottom
U$42  [#_29#ADC3#0]  25.02,31.75 0 bottom
U$43  [#LED#0]  27.94,6.35 0 bottom
U$44  [RST0]  10.16,76.2 0 top
U$45  [CS0]  10.16,74.17 0 top
U$47  [#_NC_#0]  22.1,36.83 0 top
U$48  [#_NC_#0]  22.1,34.29 0 top
U$49  [#_2#SCK#0]  25.02,39.37 0 bottom
U$50  [#_3#COPI#0]  25.15,41.91 0 bottom
U$51  [#_4#CIPO#0]  25.02,44.45 0 bottom
U$52  [#_1#RX#0]  25.02,46.99 0 bottom
U$53  [#_0#TX#0]  25.02,49.53 0 bottom
U$54  [250]  15.24,34.29 0 top
U$55  [CHARGE0]  15.24,31.75 0 top
U$56  [BOOT0]  15.24,13.97 0 top
U$57  [#22_#0]  5.46,46.99 0 bottom
U$58  [#21_#0]  5.46,44.45 0 bottom
U$59  [#20_#0]  5.46,41.91 0 bottom
U$60  [CIPO0]  10.16,70.48 0 top
U$61  [#19_#0]  5.46,39.37 0 bottom
U$62  [#18_#0]  5.46,36.83 0 bottom
U$63  [#17_#0]  5.46,34.29 0 bottom
U$64  [QWIIC_4MM]  6.73,9.4 270 top
U$65  [#16_#0]  5.46,31.75 0 bottom
U$66  [#VUSB_#0]  5.46,29.21 0 bottom
U$67  [#EN_#0]  5.46,26.67 0 bottom
U$68  [#VBATT_#0]  5.46,24.13 0 bottom
U$69  [#_NC#0]  25.02,34.29 0 bottom
U$70  [#_NC#0]  25.02,36.83 0 bottom
U$71  [#_WS2812#0]  25.02,52.07 0 bottom
U$72  [#I2C#0]  10.03,7.62 90 bottom
U$73  20.95,91.44 0 top
U$74  [SCK0]  10.16,72.39 0 top
U$75  [COPI0]  10.16,68.58 0 top
U$76  [3#3V0]  10.16,66.8 0 top
U$77  [GND0]  10.16,64.77 0 top
U$78  [GND0]  15.88,64.77 0 top
U$79  [5V0]  15.88,66.67 0 top
U$80  [SDA0]  15.88,68.58 0 top
U$81  [SCL0]  15.88,70.48 0 top
U$82  [TX0]  15.88,72.39 0 top
U$83  [RX0]  15.88,74.3 0 top
U$84  [INT0]  15.88,76.2 0 top
U$85  [PWM0]  15.88,78.11 0 top
U$88  [MIKROBUS0]  22.35,67.06 0 bottom
Y2  9.27,44.45 270 top

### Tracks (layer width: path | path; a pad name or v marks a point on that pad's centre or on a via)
1.1V  (via drill 0.2 pad 0.45)
  Top 0.127: C26.1 | C25.1 | C24.1 22.31,47.88
  Top 0.203: C25.1 22.35,44.6 20.68,42.93 20.68,42.01 20.17,41.51 U5.45 18.77,41.51 18.54,41.27 18.29,41.27 17.91,41.66 17.91,42.55 v18.41,43.05 18.87,43.51 U5.50 20.29,43.51 21.43,44.65 21.43,47 22.31,47.88 | v13.34,42.93 13.12,42.71 U5.23 11.72,42.71 11.51,42.49 11.51,41.5 10.96,40.95 10.96,40.67 C26.1
  pwrhorz 0.203: v18.41,43.05 18.29,42.93 v13.34,42.93
3.3V  (via drill 0.2 pad 0.45)
  Top 0.127: C17.1 9.84,40.42 | C22.1 18.48,49.34 | J3.2 3.56,9.9 v3.56,9.91 | 20.64,21.27 U7.5 | C3.1 14.32,52.87 v14.32,53.21 D5.VCC | C18.1 R7.2 | v16.54,50.54 v16.55,50.53
  Top 0.203: C23.1 14.88,49.51 v14.88,47.88 14.88,46.75 U5.10 | U5.49 20.02,43.11 | 20.02,43.11 20.37,43.11 21.83,44.56 21.83,45.67 C21.1 | U5.22 11.61,43.11 11.18,42.67 11.18,41.71 v10.49,41.02 10.44,41.02 9.84,40.42 | U5.1 v18.48,47.88 18.48,49.34 | U5.33 14.88,38.98 | 14.88,38.98 v14.88,38.48 | U5.44 20.43,41.11 21.18,41.86 21.18,42.52 v21.2,42.53 22.29,43.62 C18.1 | C20.1 21.01,40.18 20.69,39.87 v20.45,39.87 U5.42 | C2.1 v16.54,50.54 | U5.48 20,42.71 | 20,42.71 v20.21,42.49 | C21.1 | C21.1 v22.35,46.98 | 20,42.71 20.02,42.73 20.02,43.11 | C27.1 14.88,38.98
  Top 0.305: U7.5 20.35,21.81 C9.1 | J7.2 v21.59,20.32 20.64,21.27 | J9.7 4.32,67.44 v4.45,67.31
  Bottom 0.127: I2C.2 v13.46,9.53 | U4.8 12.59,36.09 v12.7,36.2 C4.1 C29.1 | R9.2 v18.64,29.54 | PWR.2 v23.38,7.62
  Bottom 0.305: J6.4 14.44,77.76 v14.5,77.7
  pour pwrhorz: 0,93.98 30.48,93.98 30.48,0 0,0
!BATT_ALERT!
  Top 0.127: U5.36 16.07,36.14 15.24,35.31 15.24,32.13 14.73,31.62 13.59,31.62 12.05,30.09 12.05,29.06 U2.5
!BOOT!  (via drill 0.2 pad 0.45)
  Top 0.127: v14.96,8.38 14.83,8.26 S1.3
  gndvert 0.127: v19.81,9.4 19.93,9.51 19.93,27.81 19.14,28.6 v18.64,28.6
  pwrhorz 0.127: v14.96,8.38 18.8,8.38 v19.81,9.4
  Bottom 0.127: v18.64,28.6 18.01,28.6 R5.2
!QSPI-CS!  (via drill 0.2 pad 0.45)
  Top 0.127: U5.56 19.31,48.48 v19.47,48.64
  gndvert 0.127: v19.47,48.64 19.47,39.72 19.8,39.4 19.8,37.7 v18.16,36.07
  Bottom 0.127: R5.1 R9.1 17.02,29.56 17.02,34.54 17.27,34.8 U4.1 18.16,34.82 v18.16,36.07
!RESET!  (via drill 0.2 pad 0.45)
  Top 0.127: J7.1 25.4,12.32 S2.3 | v13.61,41.62 13.5,41.51 U5.26
  gndvert 0.127: v12.7,13.97 12.7,29.84 J1.10 10.79,31.83 13.31,34.35 13.31,41.32 v13.61,41.62
  pwrhorz 0.127: J7.1 v12.7,13.97
  Bottom 0.127: J1.10 11.43,31.11 TP3.1
!SPI0_CS!  (via drill 0.2 pad 0.45)
  Top 0.127: U5.7 16.07,47.67 17.4,49 17.4,50.3 18.59,51.49 v18.59,57.01 | v18.59,73.28 11.43,73.28 7.11,77.6 J9.3
  Bottom 0.127: v18.59,57.01 v18.59,73.28
ADC0  (via drill 0.2 pad 0.45)
  Top 0.127: U5.38 16.86,39.85 16.86,36.25 18.56,34.54 22.37,34.54 22.86,34.06 22.86,24.64 23.27,24.23 v29.82,24.23 25.5,24.23 J7.5 | J9.1 23.96,82.68 v24.13,82.85
  gndvert 0.127: v24.13,82.85 24.13,59.86 30.02,53.98 30.02,24.43 v29.82,24.23
ADC1
  Top 0.127: U5.39 17.27,36.19 18.67,34.8 22.58,34.8 23.1,34.28 23.1,27.47 23.9,26.67 J7.6
ADC2
  Top 0.127: U5.40 17.68,39.22 19.2,37.7 22.66,37.7 23.36,37 23.36,29.85 24,29.21 J7.7
ADC3
  Top 0.127: U5.41 18.07,39.2 19.29,37.98 22.86,37.98 23.69,37.15 23.69,32.26 24.2,31.75 J7.8
AVDD  (via drill 0.2 pad 0.45)
  Top 0.127: U5.43 21.15,40.71 21.54,41.1 C28.1 22.36,41.66 22.61,41.91 23.11,41.91 23.37,42.16 R7.1 | v23.99,42.74 23.96,42.71 R7.1 | R7.1
  gndvert 0.127: v23.99,42.74 23.99,42.61 24,42.6 24,20.07 25.02,19.05 J7.3
EN  (via drill 0.2 pad 0.45)
  Top 0.127: U7.3 v16.76,19.37 16.32,19.37 R16.1
  Bottom 0.127: J8.2 6.22,26.67 13.34,19.56 16.58,19.56 v16.76,19.37
GND  (via drill 0.2 pad 0.45)
  Top 0.102: C8.2 16.86,22.6 v16.89,22.63
  Top 0.254: U2.4 11.93,25.9 C1.2
  other vias: 10.41,42.29 17.02,41.02 13.34,43.56 10.92,46.99 22.86,49.53 24.38,45.72 19.43,39.24 22.86,39.37 13.87,36.78 27.35,38.24 24.36,43.56 16.49,52.45 16.2,56.17 3.81,40.16 11.4,44.75 27.84,27.02 18.16,24.79 26.32,35.51 18.16,36.98 8.64,34.95 11.81,24.92 11.18,27.94 18.92,20.35 16.76,20.35 18.54,18.57 6.6,46.61 9.27,28.37 18.54,13.36 3.56,10.95 2.67,10.95 3.56,11.84 4.06,17.04 4.06,17.81 4.06,16.28 11.3,6.88 18.41,7.26 8.76,4.09 21.72,3.96 20.7,4.98 9.78,5.23 13.21,28.19 14.61,42.04 14.61,44.45 17.14,43.94 17.14,42.04 15.75,42.04 15.75,43.43 15.75,44.58
  pour gndvert: 0,93.98 30.45,93.98 30.45,0 0,0
  pour Bottom: 0,93.98 30.45,93.98 30.45,0 0,0
  pour Top: 0,93.98 30.48,93.98 30.48,0 0,0
GPIO13  (via drill 0.2 pad 0.45)
  Top 0.127: v5.94,80.01 5.81,80.14 J9.2 | v7.24,64.14 7.24,51.69 11.43,47.5 11.43,45.85 11.77,45.51 U5.16
  gndvert 0.127: v7.24,64.14 7.24,79.44 6.66,80.01 v5.94,80.01
GPIO16  (via drill 0.2 pad 0.45)
  Top 0.127: U5.27 11.91,41.11 11.59,40.79 11.59,40.04 v11.43,39.88 | v6.99,32.64 6.1,31.75 J8.4 | J9.16 25.65,82.68 24.89,81.92 v7.73,81.92
  gndvert 0.127: v7.73,81.92 7.86,81.79 7.86,39.75 v7.68,39.58 7.68,33.34 v6.99,32.64
  pwrhorz 0.127: v11.43,39.88 11.13,39.58 v7.68,39.58
GPIO17  (via drill 0.2 pad 0.45)
  Top 0.127: U5.28 12.44,40.56 v12.06,40.19 | J8.5 6.28,34.29 7.18,35.2 v7.18,40.08 | J9.15 8.63,80.14 7.32,78.83 v6.67,78.83
  gndvert 0.127: v6.67,78.83 6.67,63.83 7.18,63.32 v7.18,40.08
  pwrhorz 0.127: v12.06,40.19 11.84,40.42 8.53,40.42 8.18,40.08 v7.18,40.08
GPIO18  (via drill 0.2 pad 0.45)
  Top 0.127: U5.29 13.28,39.18 v14.1,38.35
  pwrhorz 0.127: v14.1,38.35 13.72,38.73 6.99,38.73 J8.6
GPIO19  (via drill 0.2 pad 0.45)
  Top 0.127: U5.30 13.68,39.41 v14.1,38.99
  pwrhorz 0.127: v14.1,38.99 5.46,38.99 J8.7
GPIO20  (via drill 0.2 pad 0.45)
  Top 0.127: U5.31 14.06,39.89 v14.06,40.66 | J8.8 v6.35,40.64
  pwrhorz 0.127: v14.06,40.66 14.05,40.65 v6.36,40.65 v6.35,40.64
GPIO21  (via drill 0.2 pad 0.45)
  Top 0.127: U5.32 14.47,40.48 v14.86,40.86
  pwrhorz 0.127: v14.86,40.86 14.7,41.02 12.85,41.02 11.07,42.8 6.73,42.8 J8.9
GPIO22  (via drill 0.2 pad 0.45)
  Top 0.127: U5.34 15.28,41.06 v15.49,41.27
  pwrhorz 0.127: v15.49,41.27 12.95,41.27 11.18,43.05 6.86,43.05 6.6,43.31 6.6,45.47 J8.10
I2C1_SCL/GPIO23  (via drill 0.2 pad 0.45)
  Top 0.127: v3.56,7.87 5.06,7.87 J3.4 | U2.7 10.93,29.71 v10.67,29.97 | U5.35 15.68,40.57 v16.13,41.02 | v15.66,45.81 15.28,46.19 U5.9 | J9.12 10.23,72.52 v10.23,72.53
  gndvert 0.127: v3.56,7.87 8.38,7.87 10.67,10.16 v10.67,29.97 10.06,30.58 3.93,30.58 3.3,31.21 3.3,48.77 4.06,49.53 J8.11 | v16.13,41.02 16.13,45.34 v15.66,45.81
  pwrhorz 0.127: v15.66,45.81 15.53,45.93 9.8,45.93 6.21,49.53 J8.11
  Bottom 0.127: v3.56,7.87 13.22,7.87 R10.1 | v10.23,72.53 4,72.53 1.91,70.43 1.91,50.16 2.54,49.53 J8.11
I2C1_SDA  (via drill 0.2 pad 0.45)
  Top 0.127: v3.56,8.89 v3.56,8.9 J3.3 | U2.8 10.43,29.55 10.31,29.67 v9.91,29.67 | U5.8 15.68,48.01 v15.4,48.28 | J9.11 11.01,69.98 10.58,69.55 v10.58,60.02
  gndvert 0.127: v3.56,8.89 7.75,8.89 9.91,11.05 9.91,27.8 | 9.91,27.8 v9.91,29.67 | J8.12 3.43,52.07 2.54,51.18 2.54,28.86 3.6,27.8 9.91,27.8
  pwrhorz 0.127: v15.4,48.28 14.39,48.28 v10.6,52.06 v10.6,52.07 J8.12
  Bottom 0.127: v3.56,8.89 J3.3 8.12,11.93 R17.1 | v10.58,60.02 10.6,60.02 v10.6,52.07
LED_BUILTIN
  Top 0.127: U5.37 16.48,36.16 16.24,35.93 D4.A
N$1
  Top 0.127: D4.C R3.2
N$2
  Bottom 0.127: I2C.3 13.61,8.48 R10.2
N$3
  Bottom 0.127: I2C.1 13.61,10.57 R17.2
N$4
  Top 0.127: R11.2 9.87,41.47 10.45,41.47 10.87,41.88 10.87,42.88 11.5,43.51 U5.21
N$5
  Top 0.127: Y2.P3 8.56,45.32 9.77,46.53 C16.2 10.54,46.61 10.79,46.35 10.79,44.2 11.08,43.91 U5.20
N$6
  Top 0.127: Y2.P1 9.96,43.48 C5.2 R11.1
N$7
  Top 0.127: R8.2 24.89,5.85 24.39,6.35 D3.C
N$9
  Top 0.127: D1.C 16.12,24.9 16.32,24.7 U3.1
N$10  (via drill 0.2 pad 0.45)
  Top 0.127: D3.A v20.95,6.35
  Bottom 0.127: v20.95,6.35 PWR.1
N$11
  Top 0.127: J5.A5 13.99,4.34 12.58,2.93 R1.1
N$12
  Top 0.127: R4.1 18.41,2.93 16.99,4.35 J5.B5
N$14
  Top 0.254: U3.5 13.49,24.7 R6.2
N$15
  Top 0.127: 16.2,21.27 16.13,21.34 | Q1.2 17.33,17.66 D2.C
  Top 0.305: C8.1 16.13,21.34 R16.2 | 16.2,21.27 U7.1 18.73,21.27 19.43,20.57 19.43,17.66 D2.C
N$17
  Top 0.127: R2.1 14.11,30.22 D1.A
QSPI-0  (via drill 0.2 pad 0.45)
  Top 0.127: U5.53 19.94,44.71 20.46,45.23 20.46,47.66 20.83,48.03 v20.83,49.15
  gndvert 0.127: v20.83,49.15 20.83,46.56 21.6,45.79 21.6,31.87 v22.35,31.11
  pwrhorz 0.127: v22.35,31.11 12.19,31.11 v11.81,31.5
  Bottom 0.127: v11.81,31.5 12.32,30.99 U4.5
QSPI-1  (via drill 0.2 pad 0.45)
  Top 0.127: U5.55 19.84,45.51 19.94,45.6 v19.94,49.15
  gndvert 0.127: v20.83,32.89 20.83,41.36 19.79,42.39 19.79,42.7 19.94,42.84 v19.94,49.15
  pwrhorz 0.127: v20.83,32.89 v18.92,32.89
  Bottom 0.127: v18.92,32.89 18.29,33.53 U4.2
QSPI-2  (via drill 0.2 pad 0.45)
  Top 0.127: U5.54 19.9,45.11 20.21,45.41 20.21,47.82 20.41,48.02 v20.41,48.64
  gndvert 0.127: v20.41,48.64 20.41,43.09 20.57,42.93 20.57,42.55 21.35,41.77 21.35,32.02 v20.95,31.62
  pwrhorz 0.127: v20.95,31.62 v18.92,31.62
  Bottom 0.127: v18.92,31.62 18.29,32.26 U4.3
QSPI-3  (via drill 0.2 pad 0.45)
  Top 0.127: v21.84,49.15 21.84,48.18 21.07,47.41 21.07,44.98 20,43.91 U5.51
  gndvert 0.127: v21.84,49.15 21.84,46.41 22.21,46.04 22.21,33.76 v22.45,33.53
  pwrhorz 0.127: v22.45,33.53 v11.81,33.53
  Bottom 0.127: v11.81,33.53 U4.7
QSPI-CLK  (via drill 0.2 pad 0.45)
  Top 0.127: U5.52 19.97,44.31 20.77,45.11 20.77,47.54 21.38,48.15 v21.38,48.73
  gndvert 0.127: v21.38,48.73 21.38,46.44 21.91,45.91 21.91,32.7 v22.35,32.26
  pwrhorz 0.127: v22.35,32.26 v11.81,32.26
  Bottom 0.127: v11.81,32.26 U4.6
SDIO_DAT1  (via drill 0.2 pad 0.45)
  Top 0.127: v11.61,48.41 12.75,48.41 13.28,47.88 U5.14
  Bottom 0.127: v11.61,48.41 11.17,48.85 11.17,76.46 10.03,77.6 J6.8
SDIO_DAT2  (via drill 0.2 pad 0.45)
  Top 0.127: U5.13 13.68,47.87 12.91,48.63 v12.91,51.23
  pwrhorz 0.127: v17.47,51.44 17.27,51.23 v12.91,51.23
  Bottom 0.127: v17.47,51.44 18.02,51.99 18.02,76.98 17.74,77.26 J6.1
SPI0_CIPO  (via drill 0.2 pad 0.45)
  Top 0.127: v16.38,45.72 16.48,45.81 U5.6 | J9.5 8.38,72.52 9.02,71.88 9.02,59.82 10.16,58.67 22.61,58.67 28.09,53.19 28.09,44.56 v28.08,44.55
  Bottom 0.102: J7.13 24.98,44.45
  Bottom 0.127: v16.38,45.72 16.43,45.67 16.43,45.34 17.32,44.45 24.98,44.45 | J7.13 27.98,44.45 v28.08,44.55
SPI0_COPI  (via drill 0.2 pad 0.45)
  Top 0.127: U5.5 16.88,45.48 v17.02,45.34 | J9.6 7.75,69.98 8.51,69.22 8.51,59.56 9.91,58.17 22.35,58.17 27.41,53.11 27.41,42.47 26.85,41.91 J7.12
  pwrhorz 0.127: v17.02,45.34 17.37,45.34 18.63,44.08 23.25,44.08 25.4,41.93 J7.12
SPI0_SCK  (via drill 0.2 pad 0.45)
  Top 0.127: v17.82,43.72 17.78,43.75 17.78,45.34 17.27,45.85 U5.4 | J9.4 8.26,75.06 9.53,73.79 9.53,60.07 10.41,59.18 22.99,59.18 28.73,53.44 28.73,40.67 27.42,39.37 J7.11
  pwrhorz 0.127: J7.11 21.66,43.12 19.11,43.12 18.52,43.72 v17.82,43.72
SPI_!CS1!/SDIO_DAT3  (via drill 0.2 pad 0.45)
  Top 0.127: U5.12 14.07,47.54 13.97,47.65 13.97,51.19 13.16,52 v12.5,52
  pwrhorz 0.127: v17.1,52.07 17.03,52 v12.5,52
  Bottom 0.127: v17.1,52.07 17.35,52.07 17.5,52.22 17.5,76.86 16.64,77.72 J6.2
SPI_CIPO1/SDIO_DAT0  (via drill 0.2 pad 0.45)
  Top 0.127: U5.15 12.44,47.49 v12.45,47.5
  Bottom 0.127: v12.45,47.5 12.45,48.45 11.7,49.19 11.7,76.82 11.14,77.38 J6.7
SPI_COPI1/SDIO_CMD  (via drill 0.2 pad 0.45)
  Top 0.127: U5.18 13.22,44.71 v13.34,44.82
  Bottom 0.127: v13.34,44.82 13.84,45.33 13.84,73.79 15.54,75.49 J6.3
SPI_SCK1/SDIO_CLK  (via drill 0.2 pad 0.45)
  Top 0.127: U5.17 12.98,45.11 v13.34,45.47
  Bottom 0.127: v13.34,45.47 13.34,75.82 13.72,76.2 13.72,77.09 13.34,77.47 J6.5
SWDCK  (via drill 0.2 pad 0.45)
  Top 0.127: U5.24 13.32,42.31 v13.34,42.29
  Bottom 0.127: 12.51,37.27 13.32,38.09 13.32,40.81 13.04,41.09 13.04,41.63 13.34,41.92 v13.34,42.29 | 12.51,37.27 J1.4 | TP1.1 7.49,28.07 7.49,37.34 8.04,37.89 11.89,37.89 12.51,37.27
SWDIO
  Top 0.127: U5.25 11.91,41.91 11.81,41.81 11.81,41.37 11.34,40.9 11.34,40.57 10.79,40.03 J1.2
  Bottom 0.127: TP2.1 8.26,30.48 7.75,30.99 7.75,37.21 8.13,37.59 10.03,37.59 J1.2
UART0_RX  (via drill 0.2 pad 0.45)
  Top 0.127: v18.29,45.3 18.13,45.47 18.12,45.47 17.68,45.91 U5.3 | J9.14 23.57,77.6 v23.48,77.5
  gndvert 0.127: v23.48,77.5 23.35,77.37 23.35,59.68 29.57,53.45 v29.57,47.09
  Bottom 0.127: v18.29,45.3 19.27,45.3 21.34,47.37 22.51,47.37 22.89,46.99 J7.14 25.5,47.09 v29.57,47.09
UART0_TX  (via drill 0.2 pad 0.45)
  Top 0.127: v18.29,45.88 18.07,46.09 U5.2 | J9.13 23.9,75.06 v23.75,74.9
  Bottom 0.127: J7.15 24.51,48.64 23.75,48.64 | 23.75,48.64 22.25,48.64 19.49,45.88 v18.29,45.88 | v23.75,74.9 23.75,48.64
USB_F_N  (via drill 0.2 pad 0.45)
  Top 0.127: v18.41,41.82 18.5,41.91 U5.46
  Bottom 0.127: R12.2 19.48,37.94 18.64,38.78 18.64,41.59 v18.41,41.82
USB_F_P  (via drill 0.2 pad 0.45)
  Top 0.127: v18.41,42.4 18.5,42.31 U5.47
  Bottom 0.127: R13.2 20.42,37.91 19.91,38.42 19.36,38.42 18.89,38.89 18.89,41.93 18.43,42.4 v18.41,42.4
USB_N  (via drill 0.2 pad 0.45)
  Top 0.127: J5.B7 14.49,6.74 14.61,6.86 15.49,6.86 | v16.51,8.98 15.49,7.96 15.49,7.37 15.49,7.36 15.49,6.86 | J5.A7 15.49,6.86
  Bottom 0.127: R12.1 19.52,36.41 19.52,36.4 19.56,36.37 19.56,12.03 v16.51,8.98
USB_P  (via drill 0.2 pad 0.45)
  Top 0.127: J5.A6 14.99,5.33 15.11,5.21 15.88,5.21 16,5.33 16,6 J5.B6 15.99,7.08 15.92,7.14 15.92,7.7 v15.9,7.72
  Bottom 0.127: v15.9,7.72 16.92,8.73 16.92,8.99 19.81,11.88 19.81,35.1 20.36,35.64 20.36,36.39 R13.1
V_BATT  (via drill 0.2 pad 0.45)
  Top 0.127: 10.93,25.9 C1.1 10.68,24.13
  Top 0.254: U3.3 17.11,26.66 | 17.05,27.4 v17.02,27.43
  Top 0.305: U2.2 10.93,26.29 | 10.93,26.29 10.93,25.9 | J8.1 10.68,24.13 | J4.2 10.67,19.03 | 10.67,19.03 13.86,19.03 15.03,17.86 Q1.3 | 17.11,26.66 C10.1 | U3.3 17.05,27.4 | v9.4,26.29 9.4,26.04 9.78,25.65 C1.1 10.68,19.04 10.67,19.03 | U2.3 11.43,26.42 11.3,26.29 10.93,26.29
  pwrhorz 0.305: v17.02,27.43 16.76,27.69 12.05,27.69 10.65,26.29 v9.4,26.29
V_USB  (via drill 0.2 pad 0.45)
  Top 0.254: U3.4 14.19,26.6 | 17.69,7.2 v17.65,7.24 | R15.2
  Top 0.305: Q1.1 18.85,15.56 D2.A | R15.2 17.45,14.22 17.13,14.54 Q1.1 | R2.2 C7.1 15.11,26.61 15.11,26.6 | Q1.1 16.13,16.56 16.13,17.91 14.48,19.56 14.48,21.72 15.49,22.73 15.49,23.62 | 14.19,26.6 13.62,27.18 v13.34,27.18 | J5.VBUS2 17.69,7.2 | v17.53,13.34 R15.2 | J5.VBUS1 12.79,7.2 v12.83,7.24 | U3.4 15.11,26.6 | 15.11,26.6 15.31,26.6 15.49,26.42 15.49,23.62 | J9.10 22.83,67.44 v22.7,67.31 | v28.88,22.82 21.75,22.82 20.95,23.62 15.49,23.62
  gndvert 0.254: 17.65,13.21 v17.53,13.34
  gndvert 0.305: v17.65,7.24 17.65,13.21 | v22.7,67.31 22.7,59.27 28.88,53.09 v28.88,22.82
  pwrhorz 0.305: v12.83,7.24 12.83,7.11 17.53,7.11 v17.65,7.24
  Bottom 0.305: v13.34,27.18 12.95,26.8 6.99,26.8 5.08,28.7 J8.3
WS2812_DI
  Top 0.127: U5.11 14.47,47.5 14.22,47.75 14.22,51.61 13.18,52.65 13.18,54.82 13.53,55.16 D5.DI
WS2812_DO  (via drill 0.2 pad 0.45)
  Top 0.127: D5.DO 16.94,54.06 v17,54
  pwrhorz 0.127: v17,54 23.47,54 J7.16

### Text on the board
Top: 1
gndvert: 2
pwrhorz: 3
Bottom: v10 | 4
tPlace: + | -
Measures: Units in inches
tDocu: Four Layer | 1.6mm FR4 | N. Poole | Revised by: Priyanka Makin

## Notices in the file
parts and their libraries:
SparkFun-Aesthetics: Licensing: Creative Commons ShareAlike 4.0 International - https://creativecommons.org/licenses/by-sa/4.0
SparkFun-Aesthetics: Released under the Creative Commons Attribution Share-Alike 4.0 License
SparkFun-Aesthetics: https://creativecommons.org/licenses/by-sa/4.0
